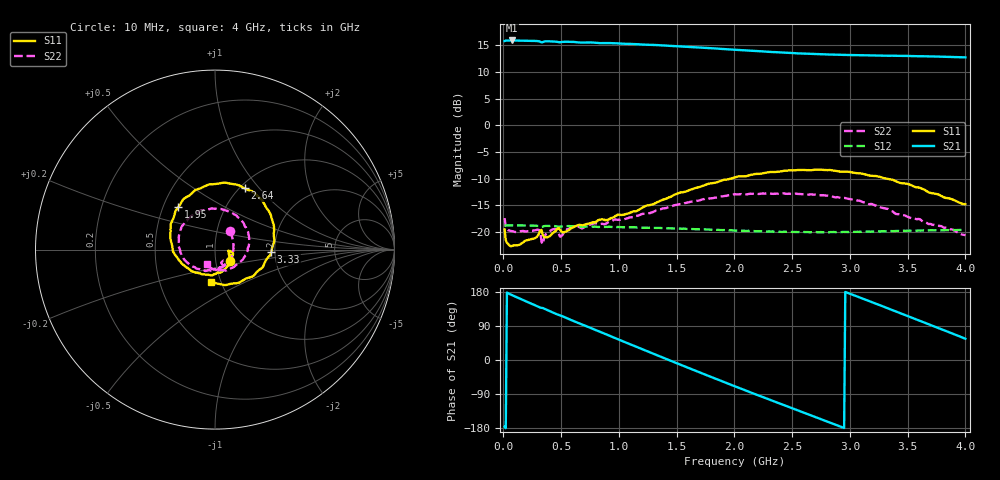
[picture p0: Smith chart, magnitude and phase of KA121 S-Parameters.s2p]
!Agilent Technologies,E5071B,JP1KK00126,A.08.11
!Date: Thu Jul 27 01:24:21 2023
!Data & Calibration Information:
!Freq	S11:SOLT2(ON)	S21:SOLT2(ON)	S12:SOLT2(ON)	S22:SOLT2(ON)
# Hz S dB R 50
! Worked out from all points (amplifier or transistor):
!   400 points, 10 MHz to 4 GHz, reference 50 ohm
!   highest |S21| = 15.9 dB at 70 MHz (marker M1)
!   |S21| within 3 dB of that: start of sweep to 3.719 GHz
!   unconditionally stable (mu >= 1): start of sweep to end of sweep
!   at 670 MHz: K = 1.08, MAG = 15.6 dB, |S12| = -19.0 dB
!   at 2.01 GHz: K = 1.14, MAG = 14.6 dB, |S12| = -19.7 dB
!   at 4 GHz: K = 1.30, MAG = 12.9 dB, |S12| = -19.7 dB
!   S11 on the Smith chart (normalised r, x): 10 MHz: 1.18, -0.15; 1.95 GHz: 0.60, +0.31; 2.64 GHz: 1.06, +0.84; 3.33 GHz: 1.91, -0.05; 4 GHz: 0.90, -0.34
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1e7  -19.54 -35.5  15.80 -176.0  -18.88 4.5  -17.40 50.5
7e7  -22.67 -6.1  15.91 171.7  -18.78 -6.4  -19.85 -3.7
2.2e8  -21.46 -5.1  15.85 151.7  -18.80 -22.3  -19.88 -35.3
4.1e8  -20.61 -20.9  15.74 127.6  -18.85 -41.3  -19.73 -60.6
5.6e8  -19.74 -36.3  15.67 108.9  -18.91 -56.0  -19.49 -76.7
6.8e8  -18.74 -54.3  15.52 93.8  -19.01 -67.9  -19.36 -90.9
9.5e8  -17.25 -90.6  15.39 60.0  -19.07 -94.7  -17.80 -113.2
1.14e9  -16.14 -120.4  15.23 36.2  -19.13 -113.6  -17.07 -129.1
1.34e9  -14.35 -151.5  15.03 11.4  -19.23 -133.4  -15.85 -146.0
1.62e9  -12.07 169.7  14.68 -23.1  -19.44 -160.8  -14.34 -174.1
1.81e9  -10.85 147.1  14.45 -46.2  -19.58 -179.0  -13.68 166.1
1.95e9  -10.11 131.0  14.24 -63.0  -19.71 167.3  -13.12 151.0
2.01e9  -9.72 124.0  14.15 -70.1  -19.73 161.7  -12.93 144.7
2.3e9  -8.79 96.0  13.77 -104.3  -19.90 134.5  -12.75 110.3
2.64e9  -8.41 63.9  13.42 -143.7  -20.03 102.9  -13.01 67.4
2.67e9  -8.42 61.0  13.38 -147.2  -20.04 100.2  -12.95 64.1
3e9  -8.75 31.2  13.18 174.9  -19.99 69.6  -13.85 21.3
3.33e9  -10.07 -2.2  13.04 136.4  -19.87 38.4  -15.69 -20.2
3.34e9  -10.11 -3.3  13.04 135.2  -19.87 37.5  -15.85 -21.7
3.5e9  -10.99 -21.0  13.00 116.2  -19.76 21.5  -17.17 -47.6
3.69e9  -12.64 -45.5  12.92 93.5  -19.71 3.0  -18.51 -75.7
4e9  -14.81 -96.9  12.74 56.1  -19.66 -28.1  -20.63 -120.5
